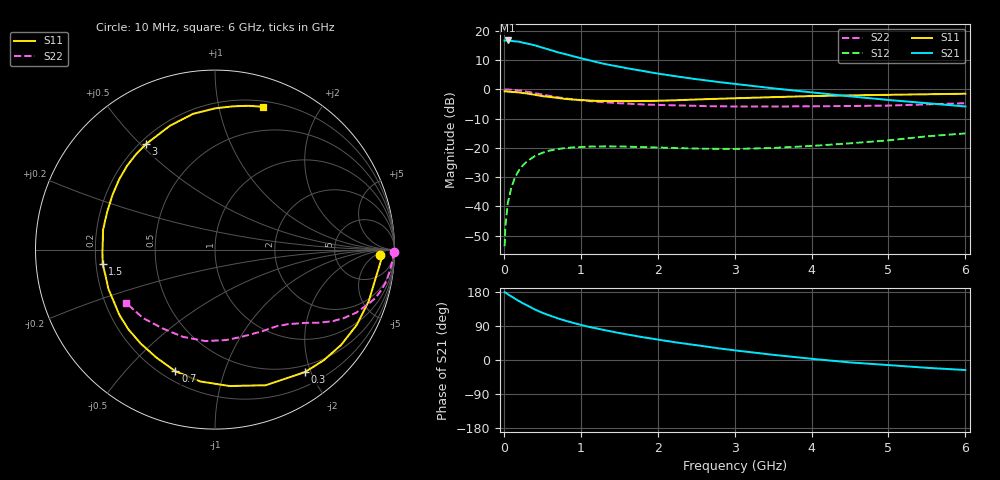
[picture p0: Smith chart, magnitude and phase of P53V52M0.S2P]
! SIEMENS Small Signal Semiconductors
! BFP183
! Si NPN RF Bipolar Junction Transistor in SOT143
! VCE = 3.5 V  IC = 2 mA
! Common Emitter S-Parameters:  March  1996
# GHz  S  MA  R  50
!  f  S11  S21  S12  S22
! GHz  MAG  ANG  MAG  ANG  MAG  ANG  MAG  ANG
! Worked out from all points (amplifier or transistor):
!   36 points, 10 MHz to 6 GHz, reference 50 ohm
!   highest |S21| = 16.7 dB at 50 MHz (marker M1)
!   |S21| within 3 dB of that: start of sweep to 572.5 MHz
!   unconditionally stable (mu >= 1): 2.102 GHz to 5.936 GHz
!   at 250 MHz: K = 0.12, MSG = 20.9 dB, |S12| = -25.9 dB
!   at 1.4 GHz: K = 0.67, MSG = 13.8 dB, |S12| = -19.5 dB
!   at 6 GHz: K = 0.99, MSG = 4.6 dB, |S12| = -15.1 dB
!   S11 on the Smith chart (normalised r, x): 10 MHz: 21, -8; 300 MHz: 0.40, -1.91; 700 MHz: 0.25, -0.70; 1.5 GHz: 0.23, -0.06; 3 GHz: 0.22, +0.52; 6 GHz: 0.25, +1.36
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0.01  0.9211 -1.9  6.777 179.0  0.0021 83.5  0.9991 -0.7
0.02  0.9269 -3.8  6.799 178.0  0.0045 85.0  0.993 -1.5
0.05  0.91 -9.6  6.813 173.7  0.0112 86.4  0.991 -3.5
0.1  0.9034 -18.5  6.685 167.5  0.0216 79.6  0.981 -7.0
0.2  0.8809 -37.1  6.489 155.1  0.0421 69.0  0.9535 -13.7
0.3  0.8467 -53.7  6.043 144.5  0.0587 60.4  0.9086 -19.3
0.4  0.8068 -69.5  5.638 133.6  0.0721 52.2  0.8611 -24.1
0.5  0.7644 -83.9  5.144 124.6  0.0825 45.0  0.8116 -28.1
0.6  0.7392 -96.4  4.707 117.1  0.0902 39.5  0.7701 -31.1
0.7  0.7129 -108.0  4.281 110.1  0.0955 34.5  0.7322 -33.5
0.8  0.6843 -118.6  3.978 103.7  0.0993 30.3  0.7004 -35.6
0.9  0.6675 -128.2  3.673 98.1  0.1019 26.7  0.6708 -37.4
1.1  0.6454 -145.6  3.158 87.7  0.105 21.1  0.6282 -40.6
1.3  0.6331 -159.8  2.728 79.3  0.106 16.8  0.6006 -43.4
1.5  0.6312 -172.7  2.426 71.2  0.1054 14.0  0.5782 -46.0
1.8  0.6333 170.0  2.064 60.4  0.1031 11.4  0.5511 -50.3
2.2  0.6473 151.9  1.696 47.6  0.0997 9.8  0.5324 -56.6
3  0.7024 123.3  1.237 25.5  0.0958 13.5  0.5084 -72.0
3.5  0.7345 109.9  1.039 13.7  0.0997 18.0  0.5078 -82.9
4.5  0.7868 90.0  0.758 -6.4  0.1196 24.0  0.5178 -110.0
5.5  0.8223 77.0  0.579 -20.6  0.1575 24.3  0.5532 -136.4
6  0.8396 71.4  0.509 -26.5  0.1764 20.9  0.5776 -149.0
